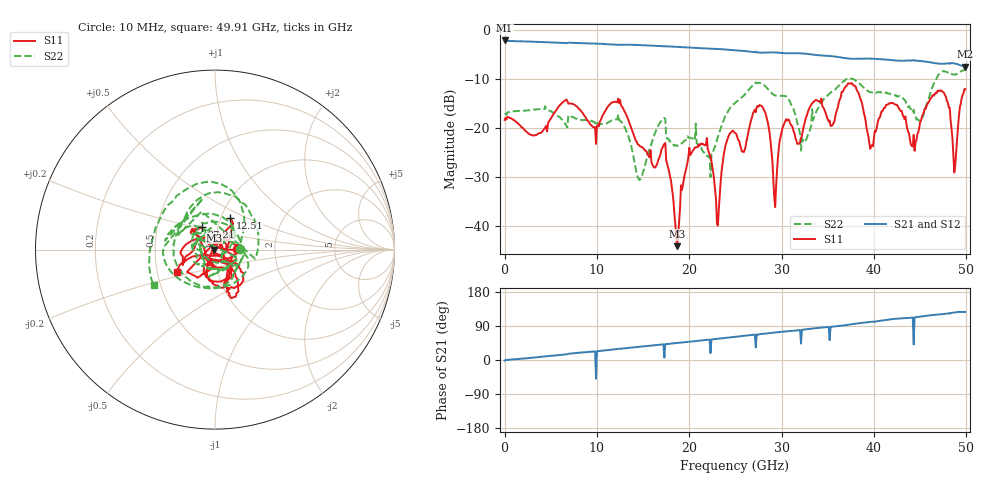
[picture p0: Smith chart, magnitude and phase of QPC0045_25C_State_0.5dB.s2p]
!File name = QPC0045_25C_State_0.5dB.s2p
!Date Time: 2024/05/06 05:46:15 AM
!Cal Ref Plane:TRL
!TEMP = 25C
!Vdd(V) = 3.15
!Vss(V) = 0.000
# GHz  S  DB  R  50
!%	Freq(GHz)  S11(dB)  S11(deg)  S21(dB)  S21(deg)  S12(dB)  S12(deg)  S22(dB)  S22(deg)
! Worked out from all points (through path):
!   500 points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, 10 MHz to 49.91 GHz, reference 50 ohm
!   highest |S21| = -2.09 dB at 10 MHz (marker M1); lowest = -7.5 dB at 49.91 GHz (marker M2)
!   lowest |S11| = -44.2 dB at 18.71 GHz (marker M3), VSWR 1.01, Z = 49.4 - j0.246 ohm
!   |S11| at or under -10 dB: start of sweep to end of sweep
!   |S22| runs from -30.7 to -8.1 dB; largest |S21 - S12| = 0.0023
!   S11 on the Smith chart (normalised r, x): 10 MHz: 1.27, +0.00; 12.51 GHz: 1.11, +0.40; 27.21 GHz: 0.84, +0.21; 49.91 GHz: 0.63, -0.17
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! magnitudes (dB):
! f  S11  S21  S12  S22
! 10 MHz  -18.4  -2.1  -2.1  -17.2
! 8.41 GHz  -16.9  -2.6  -2.6  -18.4
! 12.51 GHz  -14.2  -3.0  -3.0  -18.5
! 14.61 GHz  -23.6  -3.0  -3.0  -30.7
! 16.71 GHz  -26.3  -3.2  -3.2  -19.3
! 18.71 GHz  -44.2  -3.4  -3.4  -23.7
! 20.11 GHz  -25.5  -3.5  -3.5  -22.0
! 22.01 GHz  -24.3  -3.7  -3.7  -25.6
! 23.11 GHz  -40.0  -3.8  -3.8  -21.9
! 25.01 GHz  -21.1  -4.1  -4.1  -14.8
! 27.21 GHz  -16.8  -4.4  -4.4  -10.7
! 28.41 GHz  -18.1  -4.6  -4.6  -11.8
! 29.31 GHz  -36.2  -4.5  -4.5  -13.4
! 30.31 GHz  -19.0  -4.7  -4.7  -13.5
! 33.31 GHz  -14.9  -4.9  -4.9  -16.2
! 37.81 GHz  -11.3  -5.9  -5.9  -10.1
! 39.71 GHz  -23.7  -5.8  -5.8  -12.7
! 41.61 GHz  -15.0  -6.1  -6.0  -12.9
! 44.21 GHz  -23.8  -6.2  -6.2  -16.8
! 47.41 GHz  -12.5  -6.9  -6.9  -8.4
! 48.81 GHz  -27.7  -6.8  -6.8  -9.1
! 49.91 GHz  -12.1  -7.5  -7.5  -8.2
